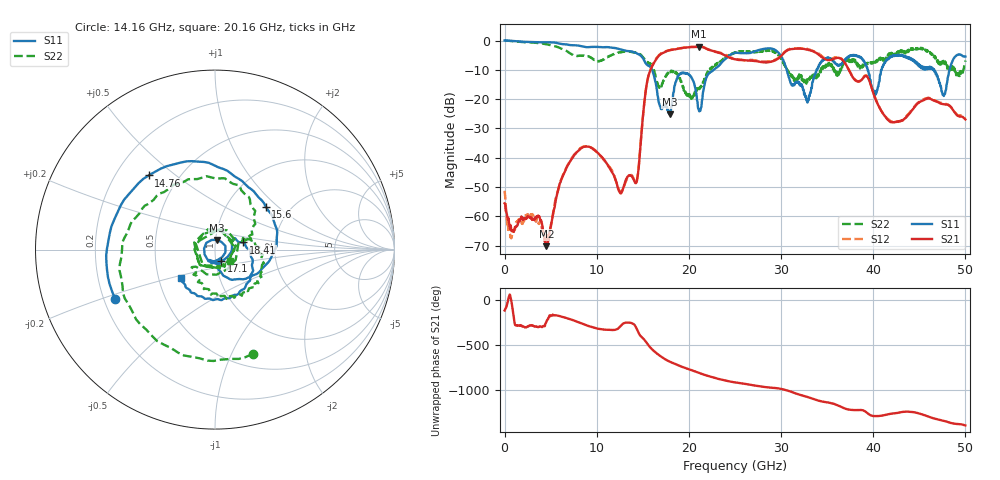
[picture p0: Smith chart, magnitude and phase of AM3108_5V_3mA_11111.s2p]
# Hz S DB R 50.0
!freq dBS11 angS11 dBS21 angS21 dBS12 angS12 dBS22 angS22
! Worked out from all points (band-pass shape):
!   1601 points, 10 MHz to 50 GHz, reference 50 ohm
!   highest |S21| = -2.14 dB at 21.13 GHz (marker M1); lowest = -70.2 dB at 4.54 GHz (marker M2)
!   |S21| within 3 dB of the highest: 16.76 GHz to 23.96 GHz (7.195 GHz wide, 35.3 % of centre); 30.05 GHz to 34.2 GHz (4.153 GHz wide, 12.9 % of centre)
!   lowest |S11| = -25.2 dB at 17.91 GHz (marker M3), VSWR 1.12, Z = 50.7 + j5.5 ohm
!   |S11| at or under -10 dB: 16 GHz to 22.68 GHz (6.683 GHz wide, 34.6 % of centre); 30.63 GHz to 33.86 GHz (3.232 GHz wide, 10 % of centre); 46.62 GHz to 48.28 GHz (1.662 GHz wide, 3.5 % of centre)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
!   |S22| runs from -19.9 to 0.0 dB; largest |S21 - S12| = 0.026
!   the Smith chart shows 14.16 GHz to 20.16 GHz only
!   S11 on the Smith chart (normalised r, x): 14.16 GHz: 0.25, -0.22; 14.76 GHz: 0.34, +0.40; 15.6 GHz: 1.51, +0.84; 17.1 GHz: 1.06, -0.13; 18.41 GHz: 1.36, +0.11; 20.16 GHz: 0.65, -0.22
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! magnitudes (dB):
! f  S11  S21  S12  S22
! 10 MHz  0.0  -55.5  -51.3  0.0
! 666.1 MHz  -0.1  -63.1  -67.0  -0.2
! 2.853 GHz  -0.5  -60.3  -59.3  -0.7
! 4.54 GHz  -0.6  -70.2  -68.9  -1.3
! 6.165 GHz  -1.2  -47.5  -47.4  -2.8
! 8.352 GHz  -2.0  -36.7  -36.4  -5.1
! 14.16 GHz  -4.1  -48.5  -48.4  -4.2
! 14.76 GHz  -5.1  -35.6  -35.3  -4.9
! 15.6 GHz  -8.6  -12.3  -12.2  -7.6
! 16.69 GHz  -20.4  -5.4  -5.2  -15.5
! 17.1 GHz  -22.9  -4.4  -4.1  -14.7
! 17.91 GHz  -25.2  -3.3  -3.3  -10.7
! 18.41 GHz  -15.9  -3.1  -2.9  -10.6
! 20.16 GHz  -12.2  -2.3  -2.2  -19.5
! 21.13 GHz  -24.2  -2.1  -2.0  -16.6
! 25 GHz  -4.2  -6.4  -6.3  -4.2
! 33.35 GHz  -15.9  -3.5  -3.4  -12.7
! 37.91 GHz  -5.0  -13.1  -13.0  -6.5
! 40.22 GHz  -18.6  -19.8  -19.6  -7.6
! 41.69 GHz  -6.1  -27.3  -27.0  -5.2
! 47.66 GHz  -18.9  -21.8  -21.5  -7.7
! 50 GHz  -5.5  -26.9  -26.5  -6.9
